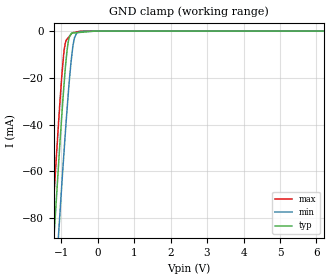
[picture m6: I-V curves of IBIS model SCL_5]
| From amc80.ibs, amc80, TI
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[Model]  SCL_5
Model_type   Input
Vinl = 0.8
Vinh = 2.0
|   typ   min   max
|   (nom PVT)   (Fast PVT)   (slow PVT)
C_comp   5.496E-13   5.421E-13   5.755E-13
| Where   nom PVT is  Nominal Process, 5.0V, 27C
|   Fast PVT is Strong Process, 5.5V, -40C
|   Slow PVT is Weak Process, 4.5V, 125C
|C_comp - from L-C Tank method, L = 1nH, peak frequency
| Where   nom PVT is  Nominal Process, 5.0V, 27C
|   Fast PVT is Strong Process, 5.5V, -40C
|   Slow PVT is Weak Process, 4.5V, 125C
|C_comp - from L-C Tank method, L = 1nH, peak frequency
[Voltage Range]   5   4.5   5.5
[Temperature Range]   27   125   -40
[Power Clamp Reference]   5   4.5   5.5
[GND Clamp Reference]   0   0   0
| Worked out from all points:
|   GND clamp passes 1 mA (typ) near -0.72 V on its own axis
[GND Clamp]
|   Voltage   I(typ)   I(min)   I(max)
-5V       -1.106A    -1.116A    -1.106A
-1.671V   -210.7mA   -237.6mA   -195.5mA
-1.249V   -101.1mA   -130.4mA   -83.83mA
-1.237V   -98.24mA   -127.4mA   -80.82mA
-1.132V   -72.19mA   -101.9mA   -54.03mA
-1.044V   -50.62mA   -80.76mA   -32.91mA
-930.8mV  -25.12mA   -53.93mA   -10.09mA
-801.9mV  -4.362mA   -26.42mA   -2.778mA
-711.4mV  -856.5uA   -10.95mA   -1.04mA
-570.9mV  -672.9uA   -767.5uA   -355.1uA
-355.4mV  -390.9uA   -3.928uA   -2.9uA
9.985V    0A         0A         0A
[POWER Clamp]
|   SCR cell for ESD function. Effects occurr above VDD x 2
|   Voltage   I(typ)   I(min)   I(max)
-5V       0A         0A         0A
0V        0A         0A         0A
10V       0A         0A         0A
